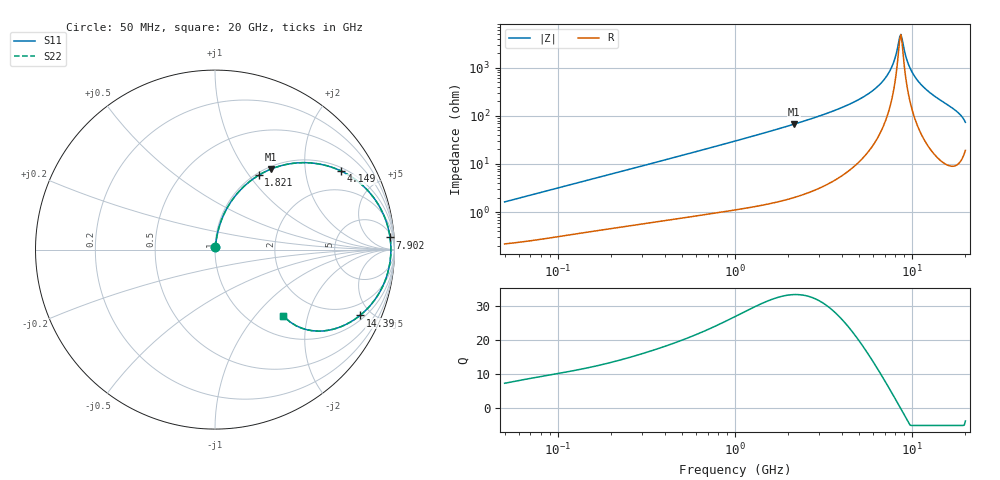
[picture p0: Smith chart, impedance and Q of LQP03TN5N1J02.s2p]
!Murata Part Number: LQP03TN5N1J02
!These Parameters are Measured in Series Mode Connection
!  o--[Z]--o
!Port1  Port2
!  o-------o
!Freq. Start=50[MHz] Stop=20[GHz], 401[Steps]
# Hz S RI R 50
!Freq.(Hz) S11(Real) S11(Imag) S21(Real) S21(Imag) S12(Real) S12(Imag) S22(Real) S22(Imag)
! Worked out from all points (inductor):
!   401 points, 50 MHz to 20 GHz, reference 50 ohm
!   read as one part in series: L = 5.11 nH near 51.52 MHz
!   highest Q = 33.5 at 2.147 GHz (marker M1), where L = 4.95 nH
!   self-resonance near 8.516 GHz
!   S11 on the Smith chart (normalised r, x): 50 MHz: 1.00, +0.03; 1.821 GHz: 1.03, +1.11; 4.149 GHz: 1.12, +3.13; 7.902 GHz: 8, +26; 14.39 GHz: 1.24, -4.28; 20 GHz: 1.38, -1.42
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5e7  0.00244 0.0161  0.9976 -0.0161  0.9976 -0.0161  0.00244 0.0161
1.364002e8  0.00546 0.0422  0.9945 -0.0422  0.9945 -0.0422  0.00546 0.0422
3.721004e8  0.0186 0.1096  0.9814 -0.1096  0.9814 -0.1096  0.0186 0.1096
1e9  0.0904 0.2688  0.9096 -0.2688  0.9096 -0.2688  0.0904 0.2688
1.820564e9  0.2437 0.4144  0.7563 -0.4144  0.7563 -0.4144  0.2437 0.4144
2.146657e9  0.314 0.4494  0.686 -0.4494  0.686 -0.4494  0.314 0.4494
2.728004e9  0.4403 0.4813  0.5597 -0.4813  0.5597 -0.4813  0.4403 0.4813
4.149438e9  0.7034 0.4375  0.2966 -0.4375  0.2966 -0.4375  0.7034 0.4375
5.944466e9  0.8985 0.2689  0.1015 -0.2689  0.1015 -0.2689  0.8985 0.2689
6.802353e9  0.9458 0.1788  0.0542 -0.1788  0.0542 -0.1788  0.9458 0.1788
7.442007e9  0.9666 0.1133  0.0334 -0.1133  0.0334 -0.1133  0.9666 0.1133
7.901521e9  0.9753 0.0679  0.0247 -0.0679  0.0247 -0.0679  0.9753 0.0679
8.389408e9  0.9796 0.0216  0.0204 -0.0216  0.0204 -0.0216  0.9796 0.0216
8.644534e9  0.9801 -0.00181  0.0199 0.00181  0.0199 0.00181  0.9801 -0.00181
8.907419e9  0.9795 -0.0252  0.0205 0.0252  0.0205 0.0252  0.9795 -0.0252
9.316812e9  0.9763 -0.0604  0.0237 0.0604  0.0237 0.0604  0.9763 -0.0604
9.600142e9  0.9728 -0.0838  0.0272 0.0838  0.0272 0.0838  0.9728 -0.0838
1.034674e10  0.9588 -0.1417  0.0412 0.1417  0.0412 0.1417  0.9588 -0.1417
1.183995e10  0.9151 -0.2414  0.0849 0.2414  0.0849 0.2414  0.9151 -0.2414
1.438523e10  0.8077 -0.367  0.1923 0.367  0.1923 0.367  0.8077 -0.367
1.800918e10  0.5863 -0.454  0.4137 0.454  0.4137 0.454  0.5863 -0.454
2e10  0.3799 -0.3687  0.6201 0.3687  0.6201 0.3687  0.3799 -0.3687
